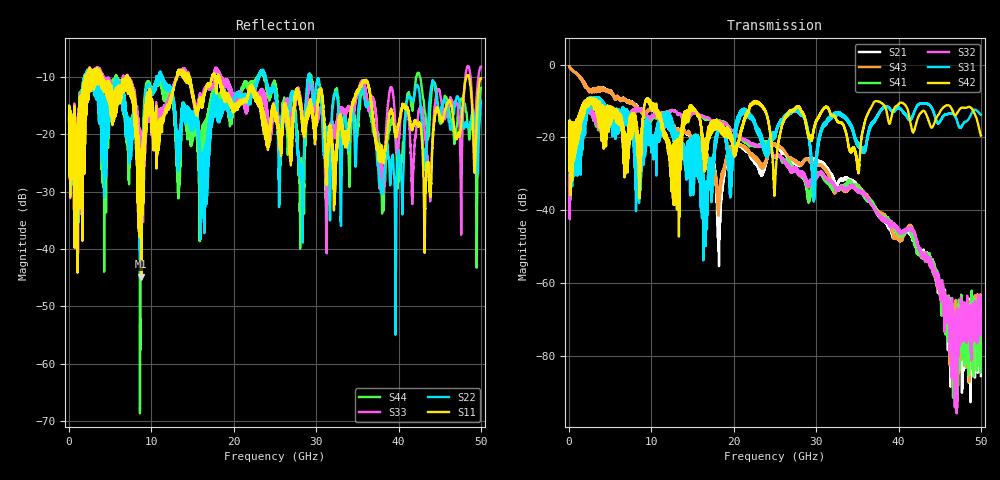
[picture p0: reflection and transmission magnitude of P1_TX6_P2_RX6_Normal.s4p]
!Keysight Technologies,N5225A,MY51441389,A.10.49.11
!Date: Monday, July 08, 2019 13:01:13
!Correction: S11(Full 4 Port(1,2,3,4))
!S12(Full 4 Port(1,2,3,4))
!S13(Full 4 Port(1,2,3,4))
!S14(Full 4 Port(1,2,3,4))
!S21(Full 4 Port(1,2,3,4))
!S22(Full 4 Port(1,2,3,4))
!S23(Full 4 Port(1,2,3,4))
!S24(Full 4 Port(1,2,3,4))
!S31(Full 4 Port(1,2,3,4))
!S32(Full 4 Port(1,2,3,4))
!S33(Full 4 Port(1,2,3,4))
!S34(Full 4 Port(1,2,3,4))
!S41(Full 4 Port(1,2,3,4))
!S42(Full 4 Port(1,2,3,4))
!S43(Full 4 Port(1,2,3,4))
!S44(Full 4 Port(1,2,3,4))
!S4P File: Measurements: <S11,S12,S13,S14>,
!<S21,S22,S23,S24>,
!<S31,S32,S33,S34>,
!<S41,S42,S43,S44>:
# Hz S  dB  R 50
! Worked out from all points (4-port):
!   5000 points, 10 MHz to 50 GHz, reference 50 ohm
!   strongest paths, dB at 10 MHz, 12.51 GHz, 25.01 GHz, 37.51 GHz, 50 GHz:
!     S42: -19.1, -27.0, -33.2, -10.1, -19.5
!     S31: -19.1, -17.9, -19.4, -13.7, -13.7
!     S32: -32.9, -12.5, -25.1, -41.3, -68.7
!     S41: -33.2, -12.4, -25.5, -40.9, -70.8
!     S43: -0.4, -16.3, -22.0, -40.4, -69.2
!     S21: -0.4, -16.2, -22.0, -41.5, -85.6
!   lowest |S11| = -44.8 dB at 8.78 GHz (marker M1), VSWR 1.01, Z = 49.5 - j0.209 ohm
!   |S11| at or under -10 dB: 4.042 GHz to 6.968 GHz (2.925 GHz wide, 53.1 % of centre); 7.073 GHz to 13.11 GHz (6.035 GHz wide, 59.8 % of centre); 18.22 GHz to 48.27 GHz (30.05 GHz wide, 90.4 % of centre)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
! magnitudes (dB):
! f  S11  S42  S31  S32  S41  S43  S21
! 10 MHz  -17.6  -19.1  -19.1  -32.9  -33.2  -0.4  -0.4
! 8.78 GHz  -44.8  -19.0  -21.7  -12.4  -12.1  -13.1  -13.0
! 9.56 GHz  -12.9  -9.9  -15.2  -14.5  -15.0  -12.6  -12.6
! 16.55 GHz  -12.5  -22.3  -39.3  -14.5  -15.1  -24.2  -24.3
! 21.17 GHz  -14.6  -16.3  -12.1  -20.6  -21.1  -22.6  -23.2
! 43.25 GHz  -32.9  -13.1  -10.6  -53.1  -53.4  -52.2  -52.1
! 50 GHz  -10.3  -19.5  -13.7  -68.7  -70.8  -69.2  -85.6
